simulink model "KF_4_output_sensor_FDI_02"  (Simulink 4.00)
settings: Solver=VariableStepDiscrete  StartTime=0.0  StopTime=100  RelTol=1e-3
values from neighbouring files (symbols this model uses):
  A = [0.9944 -0.1203 -0.4302    [process_model02.m]
  Akf1 = A - Kkf1 * C(1,:)    [UIO_KF_designs.m]
  Akf2 = A - Kkf2 * C(2,:)    [UIO_KF_designs.m]
  B = [1 0    [process_model02.m]
  Bkf1 = [B Kkf1]    [UIO_KF_designs.m]
  Bkf2 = [B Kkf2]    [UIO_KF_designs.m]
  C = [1 0 0    [process_model02.m]
  Ckf1 = C(1,:)    [UIO_KF_designs.m]
  Ckf2 = C(2,:)    [UIO_KF_designs.m]
  D = zeros(2,2)    [process_model02.m]
  Dkf1 = zeros(1,3)    [UIO_KF_designs.m]
  Dkf2 = zeros(1,3)    [UIO_KF_designs.m]
  q1 = (0.1)^2    (= 0.01)    [process_model02.m]    (also in UIO_KF_designs.m)
  q2 = (0.05)^2    (= 0.0025)    [process_model02.m]    (also in UIO_KF_designs.m)
  r1 = (7)^2    (= 49)    [process_model02.m]    (also in UIO_KF_designs.m)
  r2 = (0.6)^2    (= 0.36)    [process_model02.m]    (also in UIO_KF_designs.m)
  Ts = 0.1    [process_model02.m]
  x0 = [0.01 0.02 0.03]    [process_model02.m]
libraries: simulink3 x2

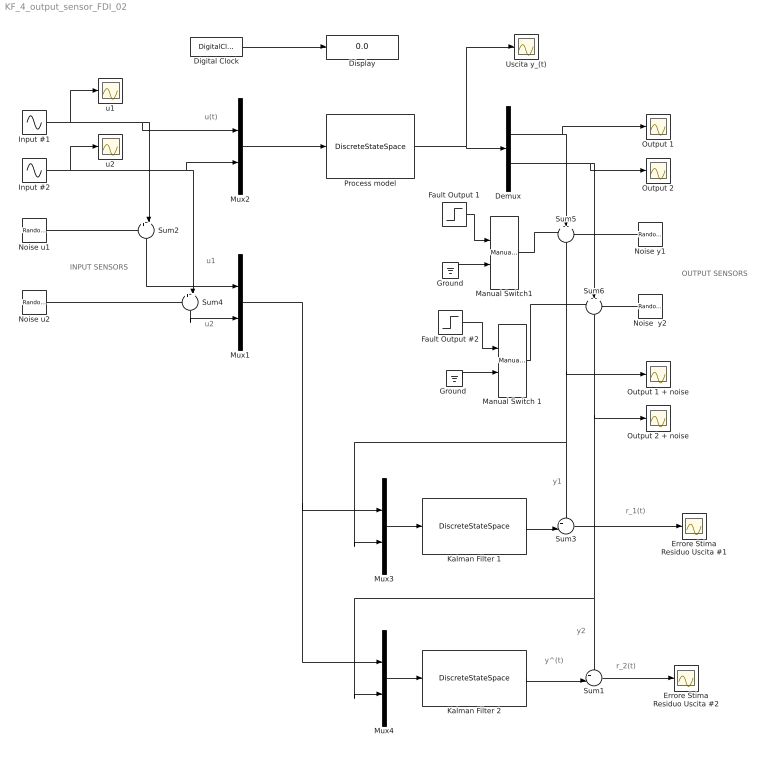
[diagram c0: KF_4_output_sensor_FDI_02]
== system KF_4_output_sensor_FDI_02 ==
  note: u(t)
  note: y^(t)
  note: r_1(t)
  note: r_2(t)
  note: INPUT SENSORS
  note: OUTPUT SENSORS
  note: u1
  note: u2
  note: y1
  note: y2
  Demux : Demux  Outputs=2  BusSelectionMode=off
  Digital Clock : DigitalClock  SampleTime=Ts
  Display : Display
  Errore Stima Residuo Uscita #1 : Scope
  Errore Stima Residuo Uscita #2 : Scope
  Fault Output #2 : Step  Time=50  Before=0  After=5  SampleTime=Ts
  Fault Output 1 : Step  Time=50  Before=0  After=100  SampleTime=Ts
  Ground : Ground
  "Ground " : Ground
  Input #1 : Sin  SineType=Time-based  Amplitude=1  Bias=0  Frequency=1  Phase=0  Samples=10  SampleTime=Ts
  Input #2 : Sin  SineType=Time-based  Amplitude=0.5  Bias=0  Frequency=0.5  Phase=pi/2  Samples=10  SampleTime=Ts
  Kalman Filter 1 : DiscreteStateSpace  A=Akf1  B=Bkf1  C=Ckf1  D=Dkf1  X0=0  SampleTime=Ts  Realization=auto
  Kalman Filter 2 : DiscreteStateSpace  A=Akf2  B=Bkf2  C=Ckf2  D=Dkf2  X0=0  SampleTime=Ts  Realization=auto
  Manual Switch 1 : simulink3/Nonlinear/Manual Switch  sw=0  action=0
  Manual Switch1 : simulink3/Nonlinear/Manual Switch  sw=0  action=0
  Mux{1..4} (4 alike) : Mux  Inputs=2
  Noise u1 : RandomNumber  Mean=0  Variance=q1  Seed=1  SampleTime=Ts
  Noise u2 : RandomNumber  Mean=0  Variance=q2  Seed=2  SampleTime=Ts
  Noise y1 : RandomNumber  Orientation=left  Mean=0  Variance=r1  Seed=3  SampleTime=Ts
  Noise  y2 : RandomNumber  Orientation=left  Mean=0  Variance=r2  Seed=4  SampleTime=Ts
  Output 1 : Scope
  Output 1 + noise : Scope
  Output 2 : Scope
  Output 2 + noise : Scope
  Process model : DiscreteStateSpace  A=A  B=B  C=C  D=D  X0=x0  SampleTime=Ts  Realization=auto
  Sum1 : Sum  Inputs=+-|  SaturateOnIntegerOverflow=on
  Sum2 : Sum  Orientation=down  Inputs=++|  SaturateOnIntegerOverflow=on
  Sum3 : Sum  Inputs=+-|  SaturateOnIntegerOverflow=on
  Sum4 : Sum  Orientation=down  Inputs=++|  SaturateOnIntegerOverflow=on
  Sum5 : Sum  Orientation=down  Inputs=+++  SaturateOnIntegerOverflow=on
  Sum6 : Sum  Orientation=down  Inputs=+++  SaturateOnIntegerOverflow=on
  Uscita y_(t) : Scope
  u1 : Scope
  u2 : Scope
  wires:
  Digital Clock/1 -> Display/1
  Mux2/1 -> Process model/1
  Input #1/1 -> u1/1, Mux2/1, Sum2/2
  Process model/1 -> Uscita y_(t)/1, Demux/1
  Sum1/1 -> Errore Stima Residuo Uscita #2/1
  Input #2/1 -> u2/1, Mux2/2, Sum4/2
  Demux/1 -> Output 1/1, Sum5/2
  Demux/2 -> Output 2/1, Sum6/2
  Ground/1 -> Manual Switch1/2
  Fault Output 1/1 -> Manual Switch1/1
  "Ground "/1 -> Manual Switch 1/2
  Fault Output #2/1 -> Manual Switch 1/1
  Manual Switch 1/1 -> Sum6/1
  Manual Switch1/1 -> Sum5/1
  Noise y1/1 -> Sum5/3
  Noise  y2/1 -> Sum6/3
  Noise u1/1 -> Sum2/1
  Noise u2/1 -> Sum4/1
  Sum2/1 -> Mux1/1
  Sum4/1 -> Mux1/2
  Mux1/1 -> Mux3/1, Mux4/1
  Sum5/1 -> Mux3/2, Sum3/1, Output 1 + noise/1
  Sum6/1 -> Mux4/2, Sum1/1, Output 2 + noise/1
  Mux4/1 -> Kalman Filter 2/1
  Mux3/1 -> Kalman Filter 1/1
  Kalman Filter 1/1 -> Sum3/2
  Sum3/1 -> Errore Stima Residuo Uscita #1/1
  Kalman Filter 2/1 -> Sum1/2
